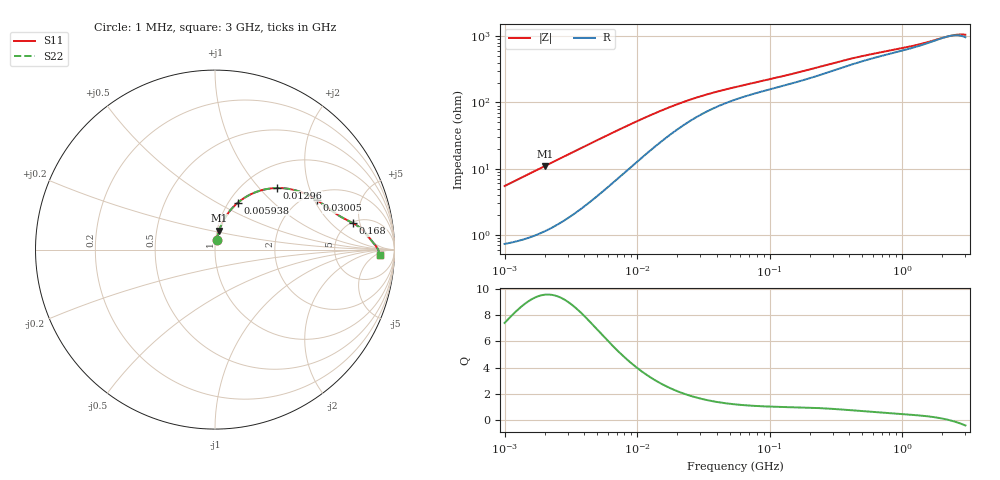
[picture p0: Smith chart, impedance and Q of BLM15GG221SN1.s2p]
! BLM15GG221SN1
# Hz S RI R 50
!Freq.(Hz) S11(Real) S11(Imag) S21(Real) S21(Imag) S12(Real) S12(Imag) S22(Real) S22(Imag)
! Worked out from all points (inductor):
!   401 points, 1 MHz to 3 GHz, reference 50 ohm
!   read as one part in series: L = 866 nH near 1.041 MHz
!   highest Q = 9.58 at 2.015 MHz (marker M1), where L = 864 nH
!   self-resonance near 2.208 GHz
!   S11 on the Smith chart (normalised r, x): 1 MHz: 1.01, +0.11; 5.938 MHz: 1.10, +0.63; 12.96 MHz: 1.40, +1.26; 30.05 MHz: 2.30, +2.11; 168 MHz: 5.18, +3.95; 3 GHz: 20, -8
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1000000  0.0102 0.0535  0.9898 -0.0535  0.9898 -0.0535  0.0102 0.0535
2014875  0.0227 0.1057  0.9773 -0.1057  0.9773 -0.1057  0.0227 0.1057
2831560  0.0382 0.145  0.9618 -0.145  0.9618 -0.145  0.0382 0.145
3823119  0.0625 0.1882  0.9375 -0.1882  0.9375 -0.1882  0.0625 0.1882
4764734  0.0897 0.2241  0.9103 -0.2241  0.9103 -0.2241  0.0897 0.2241
5938264  0.1273 0.2613  0.8727 -0.2613  0.8727 -0.2613  0.1273 0.2613
7400828  0.1768 0.2962  0.8232 -0.2962  0.8232 -0.2962  0.1768 0.2962
9223615  0.2375 0.324  0.7625 -0.324  0.7625 -0.324  0.2375 0.324
1.29622e7  0.3454 0.3431  0.6546 -0.3431  0.6546 -0.3431  0.3454 0.3431
1.461624e7  0.3842 0.3418  0.6158 -0.3418  0.6158 -0.3418  0.3842 0.3418
2.137957e7  0.4948 0.3144  0.5052 -0.3144  0.5052 -0.3144  0.4948 0.3144
3.00453e7  0.5693 0.2748  0.4307 -0.2748  0.4307 -0.2748  0.5693 0.2748
3.976269e7  0.6147 0.2429  0.3853 -0.2429  0.3853 -0.2429  0.6147 0.2429
5.477226e7  0.6553 0.2127  0.3447 -0.2127  0.3447 -0.2127  0.6553 0.2127
1.680187e8  0.7702 0.1467  0.2298 -0.1467  0.2298 -0.1467  0.7702 0.1467
2.094008e8  0.791 0.1344  0.209 -0.1344  0.209 -0.1344  0.791 0.1344
3.817355e8  0.836 0.0963  0.164 -0.0963  0.164 -0.0963  0.836 0.0963
8.005644e8  0.8674 0.0558  0.1326 -0.0558  0.1326 -0.0558  0.8674 0.0558
1.294266e9  0.8851 0.0344  0.1149 -0.0344  0.1149 -0.0344  0.8851 0.0344
2.359433e9  0.9111 -0.00606  0.0889 0.00606  0.0889 0.00606  0.9111 -0.00606
2.660507e9  0.9155 -0.0183  0.0845 0.0183  0.0845 0.0183  0.9155 -0.0183
3e9  0.9188 -0.0323  0.0812 0.0323  0.0812 0.0323  0.9188 -0.0323
